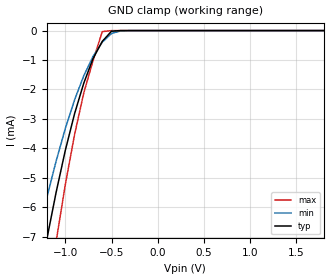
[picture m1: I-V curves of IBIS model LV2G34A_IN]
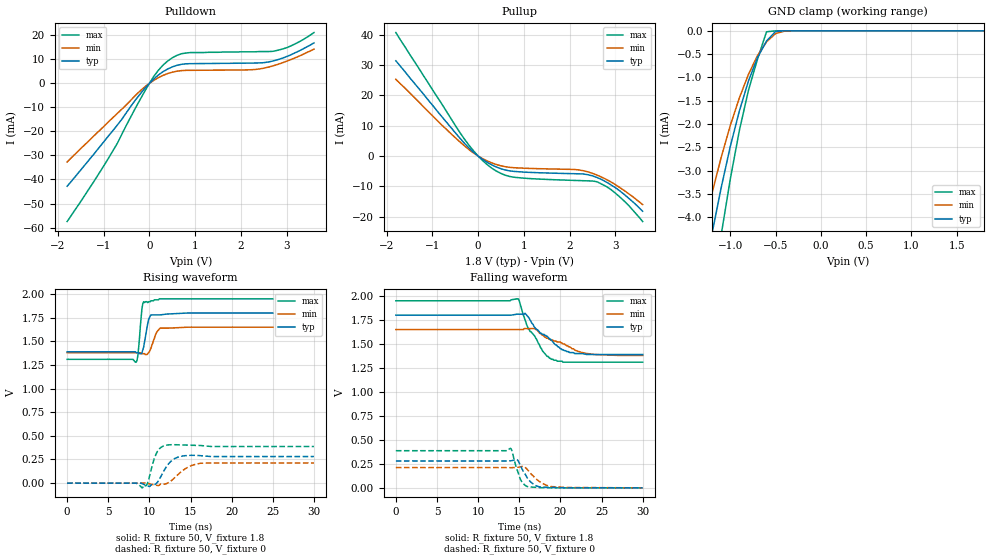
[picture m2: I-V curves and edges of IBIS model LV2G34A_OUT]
|/_/_/_/_/_/_/_/_/_/_/_/_/_/_/_/_/_/_/_/_/_/_/_/_/_/_/_/_/_/_/_/_/_/_/_/_/_/
|   Renesas Electronics Corp.
|   Multi Purpose Semiconductor Digital IC Design Group
|   IBIS Model of HD74LV2G34A
|   1.8V Triple Noninverters,  SSOP-8(8pin) Package
|   History
|   V1.0   April   1, 2003   : First release.
|/_/_/_/_/_/_/_/_/_/_/_/_/_/_/_/_/_/_/_/_/_/_/_/_/_/_/_/_/_/_/_/_/_/_/_/_/_/
[IBIS Ver]   2.1
[Comment Char]  |_char
[File name]   l2g34s1.ibs
[File Rev]   1.1
[Date]   April 1, 2003
[Source]   Data created from SPICE simulations at
|   Renesas Electronics Corp.
[Notes]   RLC value of the Package is determined by assuming typical
|   conditions.
[Disclaimer]   This information is for modeling purposes only, and is not
|   guaranteed.
[Copyright]   Copyright 2003, Renesas Electronics Corp.,
|   All Rights Reserved.
|   Component  HD74LV2G34A
[Component]   HD74LV2G34A
[Manufacturer]  Renesas Electronics Corp.
[Package]
|   typ   min   max
R_pkg   0.099   0.095   0.102
L_pkg   1.740nH   1.680nH   1.790nH
C_pkg   0.140pF   0.140pF   0.150pF
[Pin]   signal_name   model_name   R_pin   L_pin   C_pin
1   1A   LV2G34A_IN   0.102   1.780nH   0.140pF
2   3Y   LV2G34A_OUT   0.097   1.710nH   0.150pF
3   2A   LV2G34A_IN   0.095   1.680nH   0.150pF
4   GND   GND   0.102   1.790nH   0.140pF
5   2Y   LV2G34A_OUT   0.101   1.790nH   0.140pF
6   3A   LV2G34A_IN   0.097   1.710nH   0.150pF
7   1Y   LV2G34A_OUT   0.097   1.710nH   0.150pF
8   VCC   POWER   0.102   1.790nH   0.140pF
| Models and submodels in the file (2): LV2G34A_IN (Input), LV2G34A_OUT (Output)
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|   Model  LV2G34A_IN
[Model]   LV2G34A_IN
Model_type  Input
Vinl = 0.54V
Vinh = 1.26V
| variable   typ   min   max
C_comp   2.35pF   2.25pF   2.45pF
| variable   typ   min   max
[Temperature range]   25   85   -40
| variable   typ   min   max
[Voltage range]   1.8V   1.65V   1.95V
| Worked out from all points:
|   GND clamp passes 1 mA (typ) near -0.71 V on its own axis
[GND Clamp]
|   Voltage   I(typ)   I(min)   I(max)
-1.8V     -19.4mA    -15.4mA    -25.6mA
-1.3V     -8.81mA    -7.02mA    -11.6mA
-1.2V     -7.07mA    -5.66mA    -9.31mA
-1.1V     -5.49mA    -4.43mA    -7.16mA
-1V       -4.06mA    -3.32mA    -5.22mA
-900mV    -2.82mA    -2.35mA    -3.53mA
-800mV    -1.78mA    -1.53mA    -2.11mA
-700mV    -950uA     -877uA     -1.02mA
-600mV    -366uA     -393uA     -35.6uA
-500mV    -21.6uA    -99uA      -429nA
-400mV    -422nA     -10.2uA    -2.45nA
1.8V      3.69pA     25.5pA     3.6pA
|   Model  LV2G34A_OUT
[Model]   LV2G34A_OUT
Model_type  Output
Polarity   Inverting
| variable   typ   min   max
C_comp   6.35pF   6.25pF   6.45pF
| variable   typ   min   max
[Temperature range]   25   85   -40
| variable   typ   min   max
[Voltage range]   1.8V   1.65V   1.95V
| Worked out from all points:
|   slope of the pulldown table from 0 to 0.27 V, typ, clamps not added: 60.6 ohm
|   slope of the pullup table from 0 to 0.27 V, typ, clamps not added: 101 ohm
|   GND clamp passes 1 mA (typ) near -0.78 V on its own axis
|   rising waveform, R_fixture 50, V_fixture 1.8: 20-80 % time 506ps typ, 667ps min, 371ps max; typ from 1.39 V to 1.8 V
|   rising waveform, R_fixture 50, V_fixture 0: 20-80 % time 1.24ns typ, 1.85ns min, 795ps max; typ from 0 V to 0.281 V
|   falling waveform, R_fixture 50, V_fixture 1.8: 20-80 % time 3.16ns typ, 4.08ns min, 2.33ns max; typ from 1.8 V to 1.39 V
|   falling waveform, R_fixture 50, V_fixture 0: 20-80 % time 1.26ns typ, 1.73ns min, 874ps max; typ from 0.28 V to 0 V
[Pullup]
|   Voltage   I(typ)   I(min)   I(max)
-1.8V     31.4mA     25.3mA     40.7mA
-400mV    5.92mA     4.69mA     7.77mA
-100mV    1.26mA     991uA      1.71mA
200mV     -2.09mA    -1.62mA    -2.86mA
500mV     -4.2mA     -3.22mA    -5.75mA
800mV     -5.08mA    -3.86mA    -7.01mA
2.1V      -5.82mA    -4.43mA    -8.04mA
2.4V      -6.15mA    -5.21mA    -8.18mA
2.6V      -7.07mA    -6.27mA    -8.47mA
2.9V      -9.44mA    -8.5mA     -11mA
3.1V      -11.5mA    -10.4mA    -13.5mA
3.6V      -18.2mA    -16mA      -21.6mA
[Pulldown]
|   Voltage   I(typ)   I(min)   I(max)
-1.8V     -42.8mA    -32.7mA    -57.5mA
-900mV    -22mA      -16.1mA    -31.3mA
-700mV    -17.3mA    -12.5mA    -24.9mA
-100mV    -2.12mA    -1.47mA    -3.28mA
100mV     1.89mA     1.29mA     2.99mA
400mV     5.95mA     4.05mA     9.28mA
600mV     7.46mA     5.03mA     11.6mA
900mV     8.17mA     5.4mA      12.8mA
2.2V      8.4mA      5.62mA     13.1mA
2.6V      8.86mA     6.72mA     13.2mA
3V        11.1mA     9.16mA     14.8mA
3.6V      16.8mA     14.2mA     21.1mA
[GND Clamp]
|   Voltage   I(typ)   I(min)   I(max)
-1.8V     -11.9mA    -9.46mA    -15.7mA
-1.3V     -5.4mA     -4.31mA    -7.13mA
-1.2V     -4.33mA    -3.47mA    -5.69mA
-1.1V     -3.36mA    -2.71mA    -4.37mA
-1V       -2.48mA    -2.03mA    -3.18mA
-900mV    -1.72mA    -1.44mA    -2.14mA
-800mV    -1.08mA    -936uA     -1.28mA
-700mV    -575uA     -533uA     -610uA
-600mV    -219uA     -237uA     -20.5uA
-500mV    -12.9uA    -58.6uA    -245nA
-400mV    -248nA     -6.13uA    -1.4nA
1.8V      1.91pA     29.2pA     1.8pA
[Ramp]
| variable   typ   min   max
dV/dt_r   0.168/1.243n   0.128/1.841n   0.232/797.6p
dV/dt_f   0.247/3.201n   0.163/4.171n   0.386/2.351n
R_load = 50ohms
[Rising Waveform]
R_fixture = 50
V_fixture = 1.8
V_fixture_min = 1.65
V_fixture_max = 1.95
C_fixture = 0p
|   Time   V(typ)   V(min)   V(max)
0s        1.39V      1.38V      1.31V
8.4ns     1.38V      1.38V      1.28V
8.6ns     1.38V      1.38V      1.35V
9.1ns     1.38V      1.37V      1.85V
9.3ns     1.44V      1.37V      1.92V
9.9ns     1.73V      1.38V      1.92V
10.2ns    1.78V      1.43V      1.93V
10.9ns    1.78V      1.6V       1.94V
11.3ns    1.78V      1.64V      1.95V
25ns      1.8V       1.65V      1.95V
[Rising Waveform]
R_fixture = 50
V_fixture = 0
C_fixture = 0p
|   Time   V(typ)   V(min)   V(max)
0s        203pV      530nV      106pV
8.4ns     203pV      530nV      106pV
9.2ns     -8.96mV    734uV      -47.3mV
9.8ns     -29.7mV    -3.12mV    5.26mV
10.5ns    -18.3mV    -17.4mV    234mV
10.9ns    1.27mV     -23.7mV    323mV
12.1ns    177mV      -4.55mV    402mV
13.5ns    276mV      92.4mV     405mV
16.2ns    290mV      210mV      398mV
30ns      281mV      213mV      387mV
[Falling Waveform]
R_fixture = 50
V_fixture = 1.8
V_fixture_min = 1.65
V_fixture_max = 1.95
C_fixture = 0p
|   Time   V(typ)   V(min)   V(max)
0s        1.8V       1.65V      1.95V
14.9ns    1.81V      1.65V      1.97V
16.1ns    1.78V      1.66V      1.66V
17.1ns    1.65V      1.65V      1.55V
17.8ns    1.6V       1.59V      1.43V
18.9ns    1.54V      1.54V      1.34V
20.2ns    1.44V      1.51V      1.32V
21.7ns    1.4V       1.44V      1.31V
24.1ns    1.39V      1.39V      1.31V
30ns      1.39V      1.38V      1.31V
[Falling Waveform]
R_fixture = 50
V_fixture = 0
C_fixture = 0p
|   Time   V(typ)   V(min)   V(max)
0s        280mV      211mV      387mV
13.6ns    280mV      211mV      387mV
13.9ns    281mV      210mV      412mV
14.1ns    284mV      210mV      388mV
14.7ns    297mV      213mV      197mV
15.1ns    241mV      218mV      96.4mV
16ns      100mV      189mV      12.8mV
17.2ns    16.8mV     81.9mV     4.29mV
18.8ns    4.33mV     13.5mV     224uV
30ns      -78.5uV    -122uV     -32.9uV
